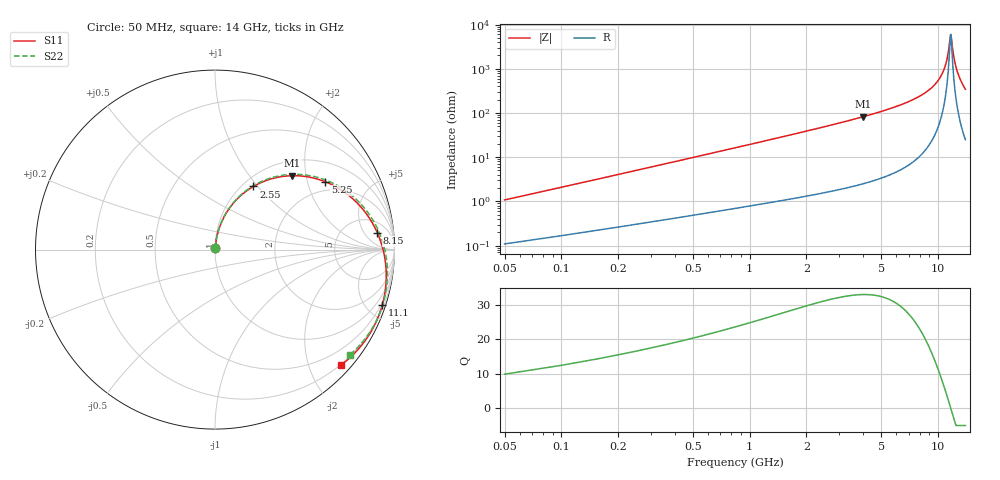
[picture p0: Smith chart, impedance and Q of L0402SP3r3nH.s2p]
!	AVX Thin Film Operation
!	Date:		5 January 2004
!	Description: 	Accu-L®  L0402 Series Thin Film RF Inductors
!	Part Number:	L04023R3BHLTR
!	50 MHz-20GHz Serial Measurements
#	mhz	S	db	R	50
!	S11	S11	S21	S21	S12	S12	S22	S22
!	dB	Phase	dB	Phase	dB	Phase	dB	Phase
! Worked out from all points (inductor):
!   280 points, 50 MHz to 14 GHz, reference 50 ohm
!   read as one part in series: L = 3.25 nH near 100 MHz
!   highest Q = 32.9 at 4 GHz (marker M1), where L = 3.26 nH
!   self-resonance near 11.7 GHz
!   S11 on the Smith chart (normalised r, x): 50 MHz: 1.00, +0.02; 2.55 GHz: 1.12, +0.95; 5.25 GHz: 1.64, +2.59; 8.15 GHz: 10, +10; 11.1 GHz: 0.36, -6.16; 14 GHz: 0.19, -2.57
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50  -40.02 83.1  -0.01 -0.7  -0.01 -0.7  -40.02 83.1
100  -34.34 83.7  -0.02 -1.3  -0.02 -1.3  -34.34 83.7
200  -28.60 83.5  -0.03 -2.5  -0.03 -2.5  -28.60 83.5
350  -23.94 82.3  -0.05 -4.3  -0.05 -4.3  -23.94 82.3
600  -19.44 79.8  -0.10 -7.2  -0.10 -7.2  -19.44 79.9
1300  -13.04 72.2  -0.30 -15.3  -0.30 -15.3  -13.04 72.5
2400  -8.17 60.3  -0.85 -27.4  -0.85 -27.4  -8.17 60.9
2550  -7.70 58.7  -0.94 -29.0  -0.94 -29.0  -7.70 59.3
4000  -4.50 43.7  -2.11 -43.9  -2.11 -43.9  -4.50 44.7
4700  -3.48 36.9  -2.84 -50.7  -2.84 -50.7  -3.48 38.0
5250  -2.84 31.6  -3.49 -55.8  -3.49 -55.8  -2.84 32.9
7050  -1.38 15.4  -6.21 -71.5  -6.21 -71.5  -1.38 17.1
8150  -0.83 5.9  -8.51 -80.3  -8.51 -80.3  -0.83 8.0
9350  -0.43 -4.1  -12.04 -89.0  -12.04 -89.0  -0.43 -1.6
10400  -0.23 -12.7  -17.09 -94.6  -17.09 -94.6  -0.23 -9.8
11100  -0.16 -18.4  -23.54 -92.9  -23.54 -92.9  -0.16 -15.2
11350  -0.15 -20.4  -27.72 -86.1  -27.72 -86.1  -0.15 -17.2
11700  -0.14 -23.3  -35.98 -23.8  -35.98 -23.8  -0.14 -19.9
12150  -0.15 -27.0  -26.00 46.3  -26.00 46.3  -0.15 -23.4
12500  -0.17 -29.9  -21.26 51.4  -21.26 51.4  -0.17 -26.1
13150  -0.25 -35.3  -16.16 50.8  -16.16 50.8  -0.25 -31.2
14000  -0.43 -42.4  -12.16 46.0  -12.16 46.0  -0.42 -37.9
